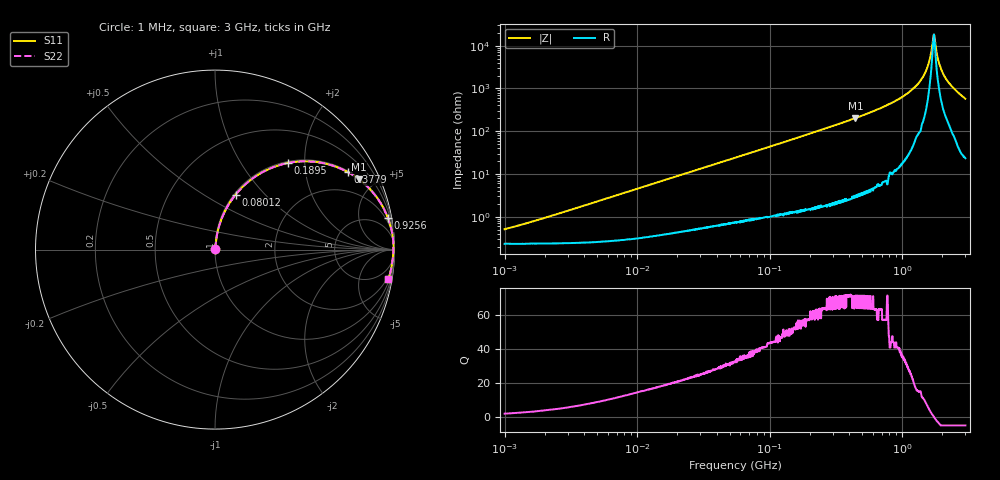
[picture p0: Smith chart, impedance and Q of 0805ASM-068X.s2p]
!s-Parameter Generated by FASTRON Sdn. Bhd.
!FASTRON P/N : 0805ASM-068X
!Keysight Technologies: E4991B_MY54100416_A.01.15
!Date: Fri Jun 19 14:49:26 2026
!Version  :Rev00  Fri Jun 19 14:49:26 2026
!Data & Calibration Information:
!Freq  S11  S21  S12  S22
!PortZ  Port1:50+j0  Port2:50+j0
!When reading reference impedance value at option line is always used.
! Remarks : This data is being provided solely for informational purposes.
# Hz S dB R 50
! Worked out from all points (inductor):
!   1601 points, 1 MHz to 3 GHz, reference 50 ohm
!   read as one part in series: L = 72.1 nH near 1.538 MHz
!   highest Q = 71.5 at 443.6 MHz (marker M1), where L = 72.6 nH
!   self-resonance near 1.73 GHz
!   S11 on the Smith chart (normalised r, x): 1 MHz: 1.00, +0.01; 80.12 MHz: 1.02, +0.70; 189.5 MHz: 1.03, +1.65; 377.9 MHz: 1.05, +3.39; 925.6 MHz: 1, +11; 3 GHz: 1, -12
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1000000  -45.90 62.7  -0.02 -0.3  -0.02 -0.3  -45.90 62.7
3804036  -35.20 80.9  -0.02 -1.0  -0.02 -1.0  -35.20 80.9
1.447069e7  -23.80 83.1  -0.05 -3.7  -0.05 -3.7  -23.80 83.1
5.504702e7  -12.70 74.8  -0.30 -13.4  -0.30 -13.4  -12.70 74.8
8.011685e7  -9.73 69.5  -0.57 -19.0  -0.57 -19.0  -9.73 69.5
1.894586e8  -4.01 49.9  -2.32 -39.1  -2.32 -39.1  -4.01 49.9
2.083556e8  -3.53 47.2  -2.68 -41.8  -2.68 -41.8  -3.53 47.2
3.779341e8  -1.35 30.3  -5.93 -58.8  -5.93 -58.8  -1.35 30.3
4.435663e8  -1.00 26.1  -7.12 -63.1  -7.12 -63.1  -1.00 26.1
7.925923e8  -0.27 13.1  -12.90 -75.7  -12.90 -75.7  -0.27 13.1
9.255909e8  -0.18 10.3  -14.90 -78.3  -14.90 -78.3  -0.18 10.3
1.159346e9  -0.09 6.4  -19.00 -81.3  -19.00 -81.3  -0.09 6.4
1.409185e9  -0.06 3.3  -24.70 -81.8  -24.70 -81.8  -0.06 3.3
1.557514e9  -0.05 1.7  -30.30 -79.1  -30.30 -79.1  -0.05 1.7
1.613037e9  -0.05 1.2  -33.60 -74.5  -33.60 -74.5  -0.05 1.2
1.695807e9  -0.05 0.4  -41.20 -50.5  -41.20 -50.5  -0.05 0.4
1.738771e9  -0.05 -0.0  -45.30 1.5  -45.30 1.5  -0.05 -0.0
1.782824e9  -0.05 -0.4  -40.80 52.0  -40.80 52.0  -0.05 -0.4
1.921792e9  -0.06 -1.6  -30.90 75.5  -30.90 75.5  -0.06 -1.6
2.092429e9  -0.07 -3.0  -25.60 79.3  -25.60 79.3  -0.07 -3.0
2.431346e9  -0.10 -5.5  -20.40 80.0  -20.40 80.0  -0.10 -5.5
3e9  -0.19 -9.8  -15.40 77.9  -15.40 77.9  -0.19 -9.8
